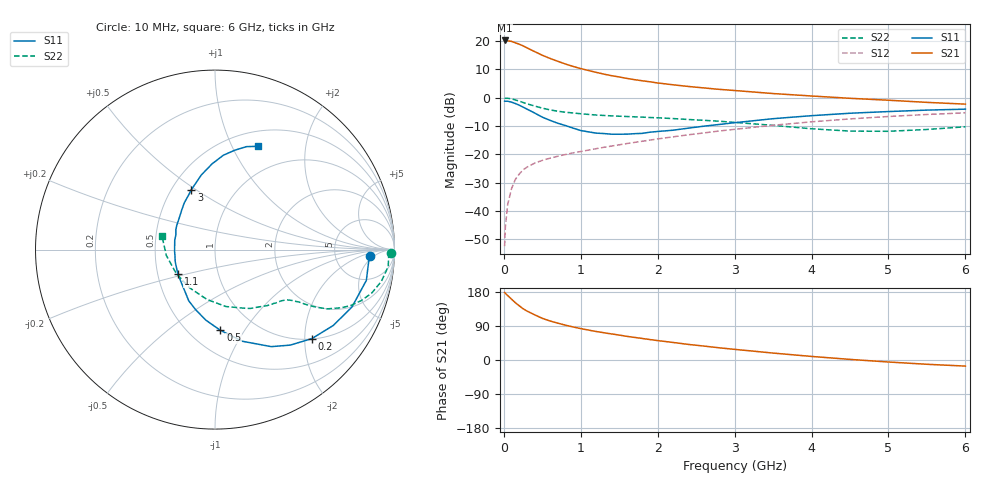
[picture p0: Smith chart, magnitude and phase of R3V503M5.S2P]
! SIEMENS Small Signal Semiconductors
! BFR181
! Si NPN RF Bipolar Junction Transistor in SOT23
! VCE = 0.5 V  IC = 3.5 mA
! Common Emitter S-Parameters:  May  1996
# GHz  S  MA  R  50
!  f  S11  S21  S12  S22
! GHz  MAG  ANG  MAG  ANG  MAG  ANG  MAG  ANG
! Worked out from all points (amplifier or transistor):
!   36 points, 10 MHz to 6 GHz, reference 50 ohm
!   highest |S21| = 20.1 dB at 10 MHz (marker M1)
!   |S21| within 3 dB of that: start of sweep to 329.8 MHz
!   unconditionally stable (mu >= 1): 914.4 MHz to 4.367 GHz
!   at 250 MHz: K = 0.40, MSG = 21.9 dB, |S12| = -25.5 dB
!   at 1.4 GHz: K = 1.16, MAG = 10.0 dB, |S12| = -17.1 dB
!   at 6 GHz: K = 0.99, MSG = 1.5 dB, |S12| = -5.4 dB
!   S11 on the Smith chart (normalised r, x): 10 MHz: 13, -4; 200 MHz: 1.01, -2.17; 500 MHz: 0.70, -0.79; 1.1 GHz: 0.64, -0.19; 3 GHz: 0.63, +0.48; 6 GHz: 0.67, +1.27
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0.01  0.8648 -2.4  10.12 178.2  0.0024 89.4  0.9786 -1.1
0.02  0.8588 -4.4  9.96 175.9  0.0053 89.9  0.9684 -2.3
0.05  0.8605 -11.5  9.958 170.1  0.013 82.9  0.9695 -5.6
0.1  0.8273 -22.8  9.762 160.6  0.0248 78.3  0.9437 -10.8
0.15  0.7827 -32.7  9.191 151.0  0.0361 71.2  0.9062 -15.5
0.2  0.7329 -42.6  8.696 143.1  0.0448 67.4  0.8634 -19.2
0.25  0.6772 -51.8  8.124 135.3  0.053 63.1  0.8177 -22.4
0.3  0.6249 -59.9  7.495 129.2  0.0592 60.8  0.7753 -24.7
0.4  0.5333 -73.3  6.449 119.3  0.0697 56.4  0.7079 -27.8
0.5  0.4507 -86.2  5.549 110.0  0.078 54.5  0.6503 -29.6
0.6  0.3963 -97.4  4.887 103.0  0.0853 53.3  0.6052 -30.8
0.8  0.3209 -117.1  3.894 92.0  0.0989 52.7  0.5504 -32.0
0.9  0.2885 -125.2  3.529 87.2  0.1058 52.9  0.5338 -32.7
1.1  0.2481 -146.2  2.992 79.0  0.1184 53.4  0.5036 -34.0
1.3  0.2317 -163.1  2.584 71.9  0.1325 54.1  0.4827 -35.5
1.6  0.2262 173.5  2.169 62.4  0.1544 54.4  0.4622 -38.6
2.2  0.2652 138.9  1.674 46.3  0.2027 53.3  0.4255 -47.3
3  0.3595 111.4  1.328 28.1  0.2748 48.8  0.3643 -63.6
3.5  0.4233 100.3  1.174 18.3  0.3241 44.6  0.3232 -79.1
4.5  0.5281 84.9  0.968 1.6  0.4197 33.2  0.2558 -123.5
5.5  0.5998 73.0  0.821 -11.3  0.5024 20.4  0.2732 -173.2
6  0.6233 67.4  0.764 -16.1  0.5366 13.5  0.305 165.6
